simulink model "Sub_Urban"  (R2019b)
settings: Solver=FixedStepAuto  StartTime=0.0  StopTime=3600*24  FixedStep=Tstep  MaxStep=1800  RelTol=1e-3
InitFcn:
  | load('network_parameters')
  | Vnom=400/sqrt(3);
  | Tstep=30*60;
  | MV_LV_transf=0;
StopFcn:
  | run('Simulink_Data.m')
undefined symbols (not defined in the file or in its folder): C_xlpe_185_90, D11, Delta, L_2x16mm, L_2x22mm, L_4x100mm, L_4x16mm, L_4x22mm, L_4x50mm, L_xlpe_185_90, LC, Line_length, R_2x16mm, R_2x22mm, R_4x100mm, R_4x16mm, R_4x22mm, R_4x50mm, R_xlpe_185_90, Source_Voltage
libraries: myLibrary x125, powerlib x89
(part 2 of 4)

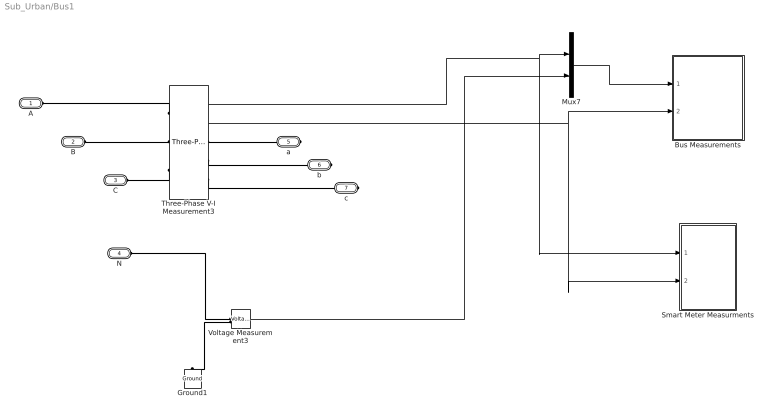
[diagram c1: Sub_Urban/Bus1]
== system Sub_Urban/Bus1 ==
  Bus Measurements : Subsystem
  Ground1 : powerlib/Elements/Ground  LConnTagsString=a
  Mux7 : Mux  Inputs=2
  Smart Meter Measurments : Subsystem
  Three-Phase V-I Measurement3 : powerlib/Measurements/Three-Phase V-I Measurement  VoltageMeasurement=phase-to-ground  SetLabelV=off  LabelV=Vabc  Vpu=off  VpuLL=off  CurrentMeasurement=yes  SetLabelI=off  LabelI=Iabc  Ipu=off  Pbase=100e6  Vbase=500e3  OutputType=Complex  PhasorSimulation=on  PSBequivalent=0
  Voltage Measurement3 : powerlib/Measurements/Voltage Measurement  PhasorSimulation=on  OutputType=Complex  PSBequivalent=0
  A : PMIOPort  Side=Left
  B : PMIOPort  Port=2  Side=Left
  C : PMIOPort  Port=3  Side=Left
  N : PMIOPort  Port=4  Side=Left
  a : PMIOPort  Port=5  Side=Right
  b : PMIOPort  Port=6  Side=Right
  c : PMIOPort  Port=7  Side=Right
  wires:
  Three-Phase V-I Measurement3/2 -> Smart Meter Measurments/2(Iabc), Bus Measurements/2(Iabc)
  Three-Phase V-I Measurement3/1 -> Smart Meter Measurments/1(Vabc), Mux7/1
  Mux7/1 -> Bus Measurements/1(Vabcn)
  Voltage Measurement3/1 -> Mux7/2
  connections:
  Three-Phase V-I Measurement3/LConn1 -- A/RConn1
  Three-Phase V-I Measurement3/LConn3 -- C/RConn1
  Three-Phase V-I Measurement3/LConn2 -- B/RConn1
  Three-Phase V-I Measurement3/RConn1 -- a/RConn1
  Three-Phase V-I Measurement3/RConn2 -- b/RConn1
  Three-Phase V-I Measurement3/RConn3 -- c/RConn1
  Voltage Measurement3/LConn1 -- N/RConn1
  Voltage Measurement3/LConn2 -- Ground1/LConn1

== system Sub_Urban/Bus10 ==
  Constant : Constant  Value=Ph
  Single Phase Load Bus : myLibrary/Single Phase Load Bus  SystemSampleTime=-1  Latency=0  AutoFrameSizeCalculation=off
  To Workspace I : ToWorkspace  VariableName=I10  SaveFormat=Structure With Time  SampleTime=-1
  To Workspace L : ToWorkspace  VariableName=Load5  SaveFormat=Structure With Time  SampleTime=-1
  To Workspace V : ToWorkspace  VariableName=Bus10  SaveFormat=Structure With Time  SampleTime=-1
  Phase : PMIOPort  Tag=PMCPort  Side=Left
  N : PMIOPort  Tag=PMCPort  Port=2  Side=Left
  phase : PMIOPort  Tag=PMCPort  Port=3  Side=Right
  n : PMIOPort  Tag=PMCPort  Port=4  Side=Right
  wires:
  Constant/1 -> Single Phase Load Bus/1
  Single Phase Load Bus/1 -> To Workspace V/1
  Single Phase Load Bus/2 -> To Workspace I/1
  Single Phase Load Bus/3 -> To Workspace L/1
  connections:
  Phase/RConn1 -- Single Phase Load Bus/LConn1
  N/RConn1 -- Single Phase Load Bus/LConn2
  phase/RConn1 -- Single Phase Load Bus/RConn1
  n/RConn1 -- Single Phase Load Bus/RConn2

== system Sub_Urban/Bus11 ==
  Constant : Constant  Value=Ph
  Single Phase Load Bus : myLibrary/Single Phase Load Bus  SystemSampleTime=-1  Latency=0  AutoFrameSizeCalculation=off
  To Workspace I : ToWorkspace  VariableName=I11  SaveFormat=Structure With Time  SampleTime=-1
  To Workspace L : ToWorkspace  VariableName=Load6  SaveFormat=Structure With Time  SampleTime=-1
  To Workspace V : ToWorkspace  VariableName=Bus11  SaveFormat=Structure With Time  SampleTime=-1
  Phase : PMIOPort  Tag=PMCPort  Side=Left
  N : PMIOPort  Tag=PMCPort  Port=2  Side=Left
  phase : PMIOPort  Tag=PMCPort  Port=3  Side=Right
  n : PMIOPort  Tag=PMCPort  Port=4  Side=Right
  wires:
  Constant/1 -> Single Phase Load Bus/1
  Single Phase Load Bus/1 -> To Workspace V/1
  Single Phase Load Bus/2 -> To Workspace I/1
  Single Phase Load Bus/3 -> To Workspace L/1
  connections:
  Phase/RConn1 -- Single Phase Load Bus/LConn1
  N/RConn1 -- Single Phase Load Bus/LConn2
  phase/RConn1 -- Single Phase Load Bus/RConn1
  n/RConn1 -- Single Phase Load Bus/RConn2

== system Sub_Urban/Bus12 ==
  Constant : Constant  Value=Ph
  Single Phase Load Bus : myLibrary/Single Phase Load Bus  SystemSampleTime=-1  Latency=0  AutoFrameSizeCalculation=off
  To Workspace I : ToWorkspace  VariableName=I12  SaveFormat=Structure With Time  SampleTime=-1
  To Workspace L : ToWorkspace  VariableName=Load7  SaveFormat=Structure With Time  SampleTime=-1
  To Workspace V : ToWorkspace  VariableName=Bus12  SaveFormat=Structure With Time  SampleTime=-1
  Phase : PMIOPort  Tag=PMCPort  Side=Left
  N : PMIOPort  Tag=PMCPort  Port=2  Side=Left
  phase : PMIOPort  Tag=PMCPort  Port=3  Side=Right
  n : PMIOPort  Tag=PMCPort  Port=4  Side=Right
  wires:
  Constant/1 -> Single Phase Load Bus/1
  Single Phase Load Bus/1 -> To Workspace V/1
  Single Phase Load Bus/2 -> To Workspace I/1
  Single Phase Load Bus/3 -> To Workspace L/1
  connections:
  Phase/RConn1 -- Single Phase Load Bus/LConn1
  N/RConn1 -- Single Phase Load Bus/LConn2
  phase/RConn1 -- Single Phase Load Bus/RConn1
  n/RConn1 -- Single Phase Load Bus/RConn2

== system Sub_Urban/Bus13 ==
  Constant : Constant  Value=Ph
  Single Phase Load Bus : myLibrary/Single Phase Load Bus  SystemSampleTime=-1  Latency=0  AutoFrameSizeCalculation=off
  To Workspace I : ToWorkspace  VariableName=I13  SaveFormat=Structure With Time  SampleTime=-1
  To Workspace L : ToWorkspace  VariableName=Load8  SaveFormat=Structure With Time  SampleTime=-1
  To Workspace V : ToWorkspace  VariableName=Bus13  SaveFormat=Structure With Time  SampleTime=-1
  Phase : PMIOPort  Tag=PMCPort  Side=Left
  N : PMIOPort  Tag=PMCPort  Port=2  Side=Left
  phase : PMIOPort  Tag=PMCPort  Port=3  Side=Right
  n : PMIOPort  Tag=PMCPort  Port=4  Side=Right
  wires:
  Constant/1 -> Single Phase Load Bus/1
  Single Phase Load Bus/1 -> To Workspace V/1
  Single Phase Load Bus/2 -> To Workspace I/1
  Single Phase Load Bus/3 -> To Workspace L/1
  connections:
  Phase/RConn1 -- Single Phase Load Bus/LConn1
  N/RConn1 -- Single Phase Load Bus/LConn2
  phase/RConn1 -- Single Phase Load Bus/RConn1
  n/RConn1 -- Single Phase Load Bus/RConn2

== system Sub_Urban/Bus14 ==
  Three Phase Zero Bus : myLibrary/Three Phase Zero Bus  SystemSampleTime=-1  Latency=0  AutoFrameSizeCalculation=off
  To Workspace I : ToWorkspace  VariableName=I14  SaveFormat=Structure With Time  SampleTime=-1
  To Workspace V : ToWorkspace  VariableName=Bus14  SaveFormat=Structure With Time  SampleTime=-1
  A : PMIOPort  Tag=PMCPort  Side=Left
  B : PMIOPort  Tag=PMCPort  Port=2  Side=Left
  C : PMIOPort  Tag=PMCPort  Port=3  Side=Left
  N : PMIOPort  Tag=PMCPort  Port=4  Side=Left
  a : PMIOPort  Tag=PMCPort  Port=5  Side=Right
  b : PMIOPort  Tag=PMCPort  Port=6  Side=Right
  c : PMIOPort  Tag=PMCPort  Port=7  Side=Right
  n : PMIOPort  Tag=PMCPort  Port=8  Side=Right
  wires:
  Three Phase Zero Bus/1 -> To Workspace V/1
  Three Phase Zero Bus/2 -> To Workspace I/1
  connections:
  A/RConn1 -- Three Phase Zero Bus/LConn1
  B/RConn1 -- Three Phase Zero Bus/LConn2
  C/RConn1 -- Three Phase Zero Bus/LConn3
  N/RConn1 -- Three Phase Zero Bus/LConn4
  a/RConn1 -- Three Phase Zero Bus/RConn1
  b/RConn1 -- Three Phase Zero Bus/RConn2
  c/RConn1 -- Three Phase Zero Bus/RConn3
  n/RConn1 -- Three Phase Zero Bus/RConn4

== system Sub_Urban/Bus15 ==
  Constant : Constant  Value=Ph
  Single Phase Load Bus : myLibrary/Single Phase Load Bus  SystemSampleTime=-1  Latency=0  AutoFrameSizeCalculation=off
  To Workspace I : ToWorkspace  VariableName=I15  SaveFormat=Structure With Time  SampleTime=-1
  To Workspace L : ToWorkspace  VariableName=Load9  SaveFormat=Structure With Time  SampleTime=-1
  To Workspace V : ToWorkspace  VariableName=Bus15  SaveFormat=Structure With Time  SampleTime=-1
  Phase : PMIOPort  Tag=PMCPort  Side=Left
  N : PMIOPort  Tag=PMCPort  Port=2  Side=Left
  phase : PMIOPort  Tag=PMCPort  Port=3  Side=Right
  n : PMIOPort  Tag=PMCPort  Port=4  Side=Right
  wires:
  Constant/1 -> Single Phase Load Bus/1
  Single Phase Load Bus/1 -> To Workspace V/1
  Single Phase Load Bus/2 -> To Workspace I/1
  Single Phase Load Bus/3 -> To Workspace L/1
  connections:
  Phase/RConn1 -- Single Phase Load Bus/LConn1
  N/RConn1 -- Single Phase Load Bus/LConn2
  phase/RConn1 -- Single Phase Load Bus/RConn1
  n/RConn1 -- Single Phase Load Bus/RConn2

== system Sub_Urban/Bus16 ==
  Three Phase Zero Bus : myLibrary/Three Phase Zero Bus  SystemSampleTime=-1  Latency=0  AutoFrameSizeCalculation=off
  To Workspace I : ToWorkspace  VariableName=I16  SaveFormat=Structure With Time  SampleTime=-1
  To Workspace V : ToWorkspace  VariableName=Bus16  SaveFormat=Structure With Time  SampleTime=-1
  A : PMIOPort  Tag=PMCPort  Side=Left
  B : PMIOPort  Tag=PMCPort  Port=2  Side=Left
  C : PMIOPort  Tag=PMCPort  Port=3  Side=Left
  N : PMIOPort  Tag=PMCPort  Port=4  Side=Left
  a : PMIOPort  Tag=PMCPort  Port=5  Side=Right
  b : PMIOPort  Tag=PMCPort  Port=6  Side=Right
  c : PMIOPort  Tag=PMCPort  Port=7  Side=Right
  n : PMIOPort  Tag=PMCPort  Port=8  Side=Right
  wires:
  Three Phase Zero Bus/1 -> To Workspace V/1
  Three Phase Zero Bus/2 -> To Workspace I/1
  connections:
  A/RConn1 -- Three Phase Zero Bus/LConn1
  B/RConn1 -- Three Phase Zero Bus/LConn2
  C/RConn1 -- Three Phase Zero Bus/LConn3
  N/RConn1 -- Three Phase Zero Bus/LConn4
  a/RConn1 -- Three Phase Zero Bus/RConn1
  b/RConn1 -- Three Phase Zero Bus/RConn2
  c/RConn1 -- Three Phase Zero Bus/RConn3
  n/RConn1 -- Three Phase Zero Bus/RConn4

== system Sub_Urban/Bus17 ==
  Constant : Constant  Value=Ph
  Single Phase Load Bus : myLibrary/Single Phase Load Bus  SystemSampleTime=-1  Latency=0  AutoFrameSizeCalculation=off
  To Workspace I : ToWorkspace  VariableName=I17  SaveFormat=Structure With Time  SampleTime=-1
  To Workspace L : ToWorkspace  VariableName=Load10  SaveFormat=Structure With Time  SampleTime=-1
  To Workspace V : ToWorkspace  VariableName=Bus17  SaveFormat=Structure With Time  SampleTime=-1
  Phase : PMIOPort  Tag=PMCPort  Side=Left
  N : PMIOPort  Tag=PMCPort  Port=2  Side=Left
  phase : PMIOPort  Tag=PMCPort  Port=3  Side=Right
  n : PMIOPort  Tag=PMCPort  Port=4  Side=Right
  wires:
  Constant/1 -> Single Phase Load Bus/1
  Single Phase Load Bus/1 -> To Workspace V/1
  Single Phase Load Bus/2 -> To Workspace I/1
  Single Phase Load Bus/3 -> To Workspace L/1
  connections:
  Phase/RConn1 -- Single Phase Load Bus/LConn1
  N/RConn1 -- Single Phase Load Bus/LConn2
  phase/RConn1 -- Single Phase Load Bus/RConn1
  n/RConn1 -- Single Phase Load Bus/RConn2

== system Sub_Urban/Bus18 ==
  Constant : Constant  Value=Ph
  Single Phase Load Bus : myLibrary/Single Phase Load Bus  SystemSampleTime=-1  Latency=0  AutoFrameSizeCalculation=off
  To Workspace I : ToWorkspace  VariableName=I18  SaveFormat=Structure With Time  SampleTime=-1
  To Workspace L : ToWorkspace  VariableName=Load11  SaveFormat=Structure With Time  SampleTime=-1
  To Workspace V : ToWorkspace  VariableName=Bus18  SaveFormat=Structure With Time  SampleTime=-1
  Phase : PMIOPort  Tag=PMCPort  Side=Left
  N : PMIOPort  Tag=PMCPort  Port=2  Side=Left
  phase : PMIOPort  Tag=PMCPort  Port=3  Side=Right
  n : PMIOPort  Tag=PMCPort  Port=4  Side=Right
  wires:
  Constant/1 -> Single Phase Load Bus/1
  Single Phase Load Bus/1 -> To Workspace V/1
  Single Phase Load Bus/2 -> To Workspace I/1
  Single Phase Load Bus/3 -> To Workspace L/1
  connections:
  Phase/RConn1 -- Single Phase Load Bus/LConn1
  N/RConn1 -- Single Phase Load Bus/LConn2
  phase/RConn1 -- Single Phase Load Bus/RConn1
  n/RConn1 -- Single Phase Load Bus/RConn2

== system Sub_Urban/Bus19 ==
  Constant : Constant  Value=Ph
  Single Phase Load Bus : myLibrary/Single Phase Load Bus  SystemSampleTime=-1  Latency=0  AutoFrameSizeCalculation=off
  To Workspace I : ToWorkspace  VariableName=I19  SaveFormat=Structure With Time  SampleTime=-1
  To Workspace L : ToWorkspace  VariableName=Load12  SaveFormat=Structure With Time  SampleTime=-1
  To Workspace V : ToWorkspace  VariableName=Bus19  SaveFormat=Structure With Time  SampleTime=-1
  Phase : PMIOPort  Tag=PMCPort  Side=Left
  N : PMIOPort  Tag=PMCPort  Port=2  Side=Left
  phase : PMIOPort  Tag=PMCPort  Port=3  Side=Right
  n : PMIOPort  Tag=PMCPort  Port=4  Side=Right
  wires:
  Constant/1 -> Single Phase Load Bus/1
  Single Phase Load Bus/1 -> To Workspace V/1
  Single Phase Load Bus/2 -> To Workspace I/1
  Single Phase Load Bus/3 -> To Workspace L/1
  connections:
  Phase/RConn1 -- Single Phase Load Bus/LConn1
  N/RConn1 -- Single Phase Load Bus/LConn2
  phase/RConn1 -- Single Phase Load Bus/RConn1
  n/RConn1 -- Single Phase Load Bus/RConn2

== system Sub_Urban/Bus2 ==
  Three Phase Zero Bus : myLibrary/Three Phase Zero Bus  SystemSampleTime=-1  Latency=0  AutoFrameSizeCalculation=off
  To Workspace I : ToWorkspace  VariableName=I2  SaveFormat=Structure With Time  SampleTime=-1
  To Workspace V : ToWorkspace  VariableName=Bus2  SaveFormat=Structure With Time  SampleTime=-1
  A : PMIOPort  Tag=PMCPort  Side=Left
  B : PMIOPort  Tag=PMCPort  Port=2  Side=Left
  C : PMIOPort  Tag=PMCPort  Port=3  Side=Left
  N : PMIOPort  Tag=PMCPort  Port=4  Side=Left
  a : PMIOPort  Tag=PMCPort  Port=5  Side=Right
  b : PMIOPort  Tag=PMCPort  Port=6  Side=Right
  c : PMIOPort  Tag=PMCPort  Port=7  Side=Right
  n : PMIOPort  Tag=PMCPort  Port=8  Side=Right
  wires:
  Three Phase Zero Bus/1 -> To Workspace V/1
  Three Phase Zero Bus/2 -> To Workspace I/1
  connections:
  Three Phase Zero Bus/LConn1 -- A/RConn1
  Three Phase Zero Bus/LConn2 -- B/RConn1
  Three Phase Zero Bus/LConn3 -- C/RConn1
  Three Phase Zero Bus/LConn4 -- N/RConn1
  Three Phase Zero Bus/RConn1 -- a/RConn1
  Three Phase Zero Bus/RConn2 -- b/RConn1
  Three Phase Zero Bus/RConn3 -- c/RConn1
  n/RConn1 -- Three Phase Zero Bus/RConn4

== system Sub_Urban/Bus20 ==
  Three Phase Zero Bus : myLibrary/Three Phase Zero Bus  SystemSampleTime=-1  Latency=0  AutoFrameSizeCalculation=off
  To Workspace I : ToWorkspace  VariableName=I20  SaveFormat=Structure With Time  SampleTime=-1
  To Workspace V : ToWorkspace  VariableName=Bus20  SaveFormat=Structure With Time  SampleTime=-1
  A : PMIOPort  Tag=PMCPort  Side=Left
  B : PMIOPort  Tag=PMCPort  Port=2  Side=Left
  C : PMIOPort  Tag=PMCPort  Port=3  Side=Left
  N : PMIOPort  Tag=PMCPort  Port=4  Side=Left
  a : PMIOPort  Tag=PMCPort  Port=5  Side=Right
  b : PMIOPort  Tag=PMCPort  Port=6  Side=Right
  c : PMIOPort  Tag=PMCPort  Port=7  Side=Right
  n : PMIOPort  Tag=PMCPort  Port=8  Side=Right
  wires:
  Three Phase Zero Bus/1 -> To Workspace V/1
  Three Phase Zero Bus/2 -> To Workspace I/1
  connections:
  A/RConn1 -- Three Phase Zero Bus/LConn1
  B/RConn1 -- Three Phase Zero Bus/LConn2
  C/RConn1 -- Three Phase Zero Bus/LConn3
  N/RConn1 -- Three Phase Zero Bus/LConn4
  a/RConn1 -- Three Phase Zero Bus/RConn1
  b/RConn1 -- Three Phase Zero Bus/RConn2
  c/RConn1 -- Three Phase Zero Bus/RConn3
  n/RConn1 -- Three Phase Zero Bus/RConn4

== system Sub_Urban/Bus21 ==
  Constant : Constant  Value=Ph
  Single Phase Load Bus : myLibrary/Single Phase Load Bus  SystemSampleTime=-1  Latency=0  AutoFrameSizeCalculation=off
  To Workspace I : ToWorkspace  VariableName=I21  SaveFormat=Structure With Time  SampleTime=-1
  To Workspace L : ToWorkspace  VariableName=Load13  SaveFormat=Structure With Time  SampleTime=-1
  To Workspace V : ToWorkspace  VariableName=Bus21  SaveFormat=Structure With Time  SampleTime=-1
  Phase : PMIOPort  Tag=PMCPort  Side=Left
  N : PMIOPort  Tag=PMCPort  Port=2  Side=Left
  phase : PMIOPort  Tag=PMCPort  Port=3  Side=Right
  n : PMIOPort  Tag=PMCPort  Port=4  Side=Right
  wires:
  Constant/1 -> Single Phase Load Bus/1
  Single Phase Load Bus/1 -> To Workspace V/1
  Single Phase Load Bus/2 -> To Workspace I/1
  Single Phase Load Bus/3 -> To Workspace L/1
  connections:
  Phase/RConn1 -- Single Phase Load Bus/LConn1
  N/RConn1 -- Single Phase Load Bus/LConn2
  phase/RConn1 -- Single Phase Load Bus/RConn1
  n/RConn1 -- Single Phase Load Bus/RConn2

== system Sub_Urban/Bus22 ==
  Three Phase Zero Bus : myLibrary/Three Phase Zero Bus  SystemSampleTime=-1  Latency=0  AutoFrameSizeCalculation=off
  To Workspace I : ToWorkspace  VariableName=I22  SaveFormat=Structure With Time  SampleTime=-1
  To Workspace V : ToWorkspace  VariableName=Bus22  SaveFormat=Structure With Time  SampleTime=-1
  A : PMIOPort  Tag=PMCPort  Side=Left
  B : PMIOPort  Tag=PMCPort  Port=2  Side=Left
  C : PMIOPort  Tag=PMCPort  Port=3  Side=Left
  N : PMIOPort  Tag=PMCPort  Port=4  Side=Left
  a : PMIOPort  Tag=PMCPort  Port=5  Side=Right
  b : PMIOPort  Tag=PMCPort  Port=6  Side=Right
  c : PMIOPort  Tag=PMCPort  Port=7  Side=Right
  n : PMIOPort  Tag=PMCPort  Port=8  Side=Right
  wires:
  Three Phase Zero Bus/1 -> To Workspace V/1
  Three Phase Zero Bus/2 -> To Workspace I/1
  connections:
  A/RConn1 -- Three Phase Zero Bus/LConn1
  B/RConn1 -- Three Phase Zero Bus/LConn2
  C/RConn1 -- Three Phase Zero Bus/LConn3
  N/RConn1 -- Three Phase Zero Bus/LConn4
  a/RConn1 -- Three Phase Zero Bus/RConn1
  b/RConn1 -- Three Phase Zero Bus/RConn2
  c/RConn1 -- Three Phase Zero Bus/RConn3
  n/RConn1 -- Three Phase Zero Bus/RConn4

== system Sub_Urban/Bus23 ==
  Constant : Constant  Value=Ph
  Single Phase Load Bus : myLibrary/Single Phase Load Bus  SystemSampleTime=-1  Latency=0  AutoFrameSizeCalculation=off
  To Workspace I : ToWorkspace  VariableName=I23  SaveFormat=Structure With Time  SampleTime=-1
  To Workspace L : ToWorkspace  VariableName=Load14  SaveFormat=Structure With Time  SampleTime=-1
  To Workspace V : ToWorkspace  VariableName=Bus23  SaveFormat=Structure With Time  SampleTime=-1
  Phase : PMIOPort  Tag=PMCPort  Side=Left
  N : PMIOPort  Tag=PMCPort  Port=2  Side=Left
  phase : PMIOPort  Tag=PMCPort  Port=3  Side=Right
  n : PMIOPort  Tag=PMCPort  Port=4  Side=Right
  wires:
  Constant/1 -> Single Phase Load Bus/1
  Single Phase Load Bus/1 -> To Workspace V/1
  Single Phase Load Bus/2 -> To Workspace I/1
  Single Phase Load Bus/3 -> To Workspace L/1
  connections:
  Phase/RConn1 -- Single Phase Load Bus/LConn1
  N/RConn1 -- Single Phase Load Bus/LConn2
  phase/RConn1 -- Single Phase Load Bus/RConn1
  n/RConn1 -- Single Phase Load Bus/RConn2

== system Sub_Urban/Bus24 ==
  Constant : Constant  Value=Ph
  Single Phase Load Bus : myLibrary/Single Phase Load Bus  SystemSampleTime=-1  Latency=0  AutoFrameSizeCalculation=off
  To Workspace I : ToWorkspace  VariableName=I24  SaveFormat=Structure With Time  SampleTime=-1
  To Workspace L : ToWorkspace  VariableName=Load15  SaveFormat=Structure With Time  SampleTime=-1
  To Workspace V : ToWorkspace  VariableName=Bus24  SaveFormat=Structure With Time  SampleTime=-1
  Phase : PMIOPort  Tag=PMCPort  Side=Left
  N : PMIOPort  Tag=PMCPort  Port=2  Side=Left
  phase : PMIOPort  Tag=PMCPort  Port=3  Side=Right
  n : PMIOPort  Tag=PMCPort  Port=4  Side=Right
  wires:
  Constant/1 -> Single Phase Load Bus/1
  Single Phase Load Bus/1 -> To Workspace V/1
  Single Phase Load Bus/2 -> To Workspace I/1
  Single Phase Load Bus/3 -> To Workspace L/1
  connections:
  Phase/RConn1 -- Single Phase Load Bus/LConn1
  N/RConn1 -- Single Phase Load Bus/LConn2
  phase/RConn1 -- Single Phase Load Bus/RConn1
  n/RConn1 -- Single Phase Load Bus/RConn2

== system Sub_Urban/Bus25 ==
  Three Phase Zero Bus : myLibrary/Three Phase Zero Bus  SystemSampleTime=-1  Latency=0  AutoFrameSizeCalculation=off
  To Workspace I : ToWorkspace  VariableName=I25  SaveFormat=Structure With Time  SampleTime=-1
  To Workspace V : ToWorkspace  VariableName=Bus25  SaveFormat=Structure With Time  SampleTime=-1
  A : PMIOPort  Tag=PMCPort  Side=Left
  B : PMIOPort  Tag=PMCPort  Port=2  Side=Left
  C : PMIOPort  Tag=PMCPort  Port=3  Side=Left
  N : PMIOPort  Tag=PMCPort  Port=4  Side=Left
  a : PMIOPort  Tag=PMCPort  Port=5  Side=Right
  b : PMIOPort  Tag=PMCPort  Port=6  Side=Right
  c : PMIOPort  Tag=PMCPort  Port=7  Side=Right
  n : PMIOPort  Tag=PMCPort  Port=8  Side=Right
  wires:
  Three Phase Zero Bus/1 -> To Workspace V/1
  Three Phase Zero Bus/2 -> To Workspace I/1
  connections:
  A/RConn1 -- Three Phase Zero Bus/LConn1
  B/RConn1 -- Three Phase Zero Bus/LConn2
  C/RConn1 -- Three Phase Zero Bus/LConn3
  N/RConn1 -- Three Phase Zero Bus/LConn4
  a/RConn1 -- Three Phase Zero Bus/RConn1
  b/RConn1 -- Three Phase Zero Bus/RConn2
  c/RConn1 -- Three Phase Zero Bus/RConn3
  n/RConn1 -- Three Phase Zero Bus/RConn4

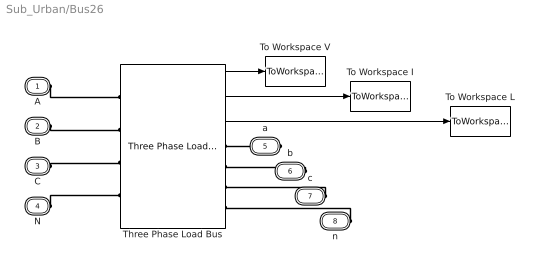
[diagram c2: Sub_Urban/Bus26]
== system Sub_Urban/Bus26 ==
  Three Phase Load Bus : myLibrary/Three Phase Load Bus  SystemSampleTime=-1  Latency=0  AutoFrameSizeCalculation=off
  To Workspace I : ToWorkspace  VariableName=I26  SaveFormat=Structure With Time  SampleTime=-1
  To Workspace L : ToWorkspace  VariableName=Load16  SaveFormat=Structure With Time  SampleTime=-1
  To Workspace V : ToWorkspace  VariableName=Bus26  SaveFormat=Structure With Time  SampleTime=-1
  A : PMIOPort  Tag=PMCPort  Side=Left
  B : PMIOPort  Tag=PMCPort  Port=2  Side=Left
  C : PMIOPort  Tag=PMCPort  Port=3  Side=Left
  N : PMIOPort  Tag=PMCPort  Port=4  Side=Left
  a : PMIOPort  Tag=PMCPort  Port=5  Side=Right
  b : PMIOPort  Tag=PMCPort  Port=6  Side=Right
  c : PMIOPort  Tag=PMCPort  Port=7  Side=Right
  n : PMIOPort  Tag=PMCPort  Port=8  Side=Right
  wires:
  Three Phase Load Bus/1 -> To Workspace V/1
  Three Phase Load Bus/2 -> To Workspace I/1
  Three Phase Load Bus/3 -> To Workspace L/1
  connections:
  N/RConn1 -- Three Phase Load Bus/LConn4
  C/RConn1 -- Three Phase Load Bus/LConn3
  n/RConn1 -- Three Phase Load Bus/RConn4
  B/RConn1 -- Three Phase Load Bus/LConn2
  A/RConn1 -- Three Phase Load Bus/LConn1
  b/RConn1 -- Three Phase Load Bus/RConn2
  c/RConn1 -- Three Phase Load Bus/RConn3
  a/RConn1 -- Three Phase Load Bus/RConn1

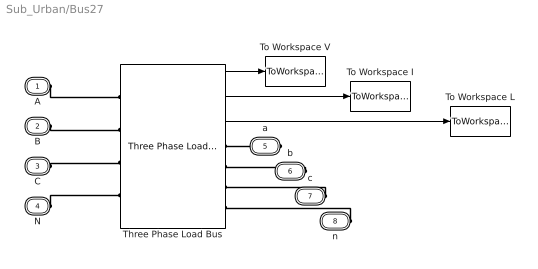
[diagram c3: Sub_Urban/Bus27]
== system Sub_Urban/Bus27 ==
  Three Phase Load Bus : myLibrary/Three Phase Load Bus  SystemSampleTime=-1  Latency=0  AutoFrameSizeCalculation=off
  To Workspace I : ToWorkspace  VariableName=I27  SaveFormat=Structure With Time  SampleTime=-1
  To Workspace L : ToWorkspace  VariableName=Load17  SaveFormat=Structure With Time  SampleTime=-1
  To Workspace V : ToWorkspace  VariableName=Bus27  SaveFormat=Structure With Time  SampleTime=-1
  A : PMIOPort  Tag=PMCPort  Side=Left
  B : PMIOPort  Tag=PMCPort  Port=2  Side=Left
  C : PMIOPort  Tag=PMCPort  Port=3  Side=Left
  N : PMIOPort  Tag=PMCPort  Port=4  Side=Left
  a : PMIOPort  Tag=PMCPort  Port=5  Side=Right
  b : PMIOPort  Tag=PMCPort  Port=6  Side=Right
  c : PMIOPort  Tag=PMCPort  Port=7  Side=Right
  n : PMIOPort  Tag=PMCPort  Port=8  Side=Right
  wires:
  Three Phase Load Bus/1 -> To Workspace V/1
  Three Phase Load Bus/2 -> To Workspace I/1
  Three Phase Load Bus/3 -> To Workspace L/1
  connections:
  N/RConn1 -- Three Phase Load Bus/LConn4
  C/RConn1 -- Three Phase Load Bus/LConn3
  n/RConn1 -- Three Phase Load Bus/RConn4
  B/RConn1 -- Three Phase Load Bus/LConn2
  A/RConn1 -- Three Phase Load Bus/LConn1
  b/RConn1 -- Three Phase Load Bus/RConn2
  c/RConn1 -- Three Phase Load Bus/RConn3
  a/RConn1 -- Three Phase Load Bus/RConn1

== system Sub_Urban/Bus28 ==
  Constant : Constant  Value=Ph
  Single Phase Load Bus : myLibrary/Single Phase Load Bus  SystemSampleTime=-1  Latency=0  AutoFrameSizeCalculation=off
  To Workspace I : ToWorkspace  VariableName=I28  SaveFormat=Structure With Time  SampleTime=-1
  To Workspace L : ToWorkspace  VariableName=Load18  SaveFormat=Structure With Time  SampleTime=-1
  To Workspace V : ToWorkspace  VariableName=Bus28  SaveFormat=Structure With Time  SampleTime=-1
  Phase : PMIOPort  Tag=PMCPort  Side=Left
  N : PMIOPort  Tag=PMCPort  Port=2  Side=Left
  phase : PMIOPort  Tag=PMCPort  Port=3  Side=Right
  n : PMIOPort  Tag=PMCPort  Port=4  Side=Right
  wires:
  Constant/1 -> Single Phase Load Bus/1
  Single Phase Load Bus/1 -> To Workspace V/1
  Single Phase Load Bus/2 -> To Workspace I/1
  Single Phase Load Bus/3 -> To Workspace L/1
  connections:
  Phase/RConn1 -- Single Phase Load Bus/LConn1
  N/RConn1 -- Single Phase Load Bus/LConn2
  phase/RConn1 -- Single Phase Load Bus/RConn1
  n/RConn1 -- Single Phase Load Bus/RConn2

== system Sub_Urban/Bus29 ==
  Constant : Constant  Value=Ph
  Single Phase Load Bus : myLibrary/Single Phase Load Bus  SystemSampleTime=-1  Latency=0  AutoFrameSizeCalculation=off
  To Workspace I : ToWorkspace  VariableName=I29  SaveFormat=Structure With Time  SampleTime=-1
  To Workspace L : ToWorkspace  VariableName=Load19  SaveFormat=Structure With Time  SampleTime=-1
  To Workspace V : ToWorkspace  VariableName=Bus29  SaveFormat=Structure With Time  SampleTime=-1
  Phase : PMIOPort  Tag=PMCPort  Side=Left
  N : PMIOPort  Tag=PMCPort  Port=2  Side=Left
  phase : PMIOPort  Tag=PMCPort  Port=3  Side=Right
  n : PMIOPort  Tag=PMCPort  Port=4  Side=Right
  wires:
  Constant/1 -> Single Phase Load Bus/1
  Single Phase Load Bus/1 -> To Workspace V/1
  Single Phase Load Bus/2 -> To Workspace I/1
  Single Phase Load Bus/3 -> To Workspace L/1
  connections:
  Phase/RConn1 -- Single Phase Load Bus/LConn1
  N/RConn1 -- Single Phase Load Bus/LConn2
  phase/RConn1 -- Single Phase Load Bus/RConn1
  n/RConn1 -- Single Phase Load Bus/RConn2

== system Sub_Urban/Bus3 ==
  Three Phase Zero Bus : myLibrary/Three Phase Zero Bus  SystemSampleTime=-1  Latency=0  AutoFrameSizeCalculation=off
  To Workspace I : ToWorkspace  VariableName=I3  SaveFormat=Structure With Time  SampleTime=-1
  To Workspace V : ToWorkspace  VariableName=Bus3  SaveFormat=Structure With Time  SampleTime=-1
  A : PMIOPort  Tag=PMCPort  Side=Left
  B : PMIOPort  Tag=PMCPort  Port=2  Side=Left
  C : PMIOPort  Tag=PMCPort  Port=3  Side=Left
  N : PMIOPort  Tag=PMCPort  Port=4  Side=Left
  a : PMIOPort  Tag=PMCPort  Port=5  Side=Right
  b : PMIOPort  Tag=PMCPort  Port=6  Side=Right
  c : PMIOPort  Tag=PMCPort  Port=7  Side=Right
  n : PMIOPort  Tag=PMCPort  Port=8  Side=Right
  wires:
  Three Phase Zero Bus/1 -> To Workspace V/1
  Three Phase Zero Bus/2 -> To Workspace I/1
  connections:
  A/RConn1 -- Three Phase Zero Bus/LConn1
  B/RConn1 -- Three Phase Zero Bus/LConn2
  C/RConn1 -- Three Phase Zero Bus/LConn3
  N/RConn1 -- Three Phase Zero Bus/LConn4
  a/RConn1 -- Three Phase Zero Bus/RConn1
  b/RConn1 -- Three Phase Zero Bus/RConn2
  c/RConn1 -- Three Phase Zero Bus/RConn3
  n/RConn1 -- Three Phase Zero Bus/RConn4

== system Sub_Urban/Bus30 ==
  Three Phase Zero Bus : myLibrary/Three Phase Zero Bus  SystemSampleTime=-1  Latency=0  AutoFrameSizeCalculation=off
  To Workspace I : ToWorkspace  VariableName=I30  SaveFormat=Structure With Time  SampleTime=-1
  To Workspace V : ToWorkspace  VariableName=Bus30  SaveFormat=Structure With Time  SampleTime=-1
  A : PMIOPort  Tag=PMCPort  Side=Left
  B : PMIOPort  Tag=PMCPort  Port=2  Side=Left
  C : PMIOPort  Tag=PMCPort  Port=3  Side=Left
  N : PMIOPort  Tag=PMCPort  Port=4  Side=Left
  a : PMIOPort  Tag=PMCPort  Port=5  Side=Right
  b : PMIOPort  Tag=PMCPort  Port=6  Side=Right
  c : PMIOPort  Tag=PMCPort  Port=7  Side=Right
  n : PMIOPort  Tag=PMCPort  Port=8  Side=Right
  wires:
  Three Phase Zero Bus/1 -> To Workspace V/1
  Three Phase Zero Bus/2 -> To Workspace I/1
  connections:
  A/RConn1 -- Three Phase Zero Bus/LConn1
  B/RConn1 -- Three Phase Zero Bus/LConn2
  C/RConn1 -- Three Phase Zero Bus/LConn3
  N/RConn1 -- Three Phase Zero Bus/LConn4
  a/RConn1 -- Three Phase Zero Bus/RConn1
  b/RConn1 -- Three Phase Zero Bus/RConn2
  c/RConn1 -- Three Phase Zero Bus/RConn3
  n/RConn1 -- Three Phase Zero Bus/RConn4

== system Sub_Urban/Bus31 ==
  Three Phase Zero Bus : myLibrary/Three Phase Zero Bus  SystemSampleTime=-1  Latency=0  AutoFrameSizeCalculation=off
  To Workspace I : ToWorkspace  VariableName=I31  SaveFormat=Structure With Time  SampleTime=-1
  To Workspace V : ToWorkspace  VariableName=Bus31  SaveFormat=Structure With Time  SampleTime=-1
  A : PMIOPort  Tag=PMCPort  Side=Left
  B : PMIOPort  Tag=PMCPort  Port=2  Side=Left
  C : PMIOPort  Tag=PMCPort  Port=3  Side=Left
  N : PMIOPort  Tag=PMCPort  Port=4  Side=Left
  a : PMIOPort  Tag=PMCPort  Port=5  Side=Right
  b : PMIOPort  Tag=PMCPort  Port=6  Side=Right
  c : PMIOPort  Tag=PMCPort  Port=7  Side=Right
  n : PMIOPort  Tag=PMCPort  Port=8  Side=Right
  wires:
  Three Phase Zero Bus/1 -> To Workspace V/1
  Three Phase Zero Bus/2 -> To Workspace I/1
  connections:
  A/RConn1 -- Three Phase Zero Bus/LConn1
  B/RConn1 -- Three Phase Zero Bus/LConn2
  C/RConn1 -- Three Phase Zero Bus/LConn3
  N/RConn1 -- Three Phase Zero Bus/LConn4
  a/RConn1 -- Three Phase Zero Bus/RConn1
  b/RConn1 -- Three Phase Zero Bus/RConn2
  c/RConn1 -- Three Phase Zero Bus/RConn3
  n/RConn1 -- Three Phase Zero Bus/RConn4

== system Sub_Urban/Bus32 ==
  Constant : Constant  Value=Ph
  Single Phase Load Bus : myLibrary/Single Phase Load Bus  SystemSampleTime=-1  Latency=0  AutoFrameSizeCalculation=off
  To Workspace I : ToWorkspace  VariableName=I32  SaveFormat=Structure With Time  SampleTime=-1
  To Workspace L : ToWorkspace  VariableName=Load20  SaveFormat=Structure With Time  SampleTime=-1
  To Workspace V : ToWorkspace  VariableName=Bus32  SaveFormat=Structure With Time  SampleTime=-1
  Phase : PMIOPort  Tag=PMCPort  Side=Left
  N : PMIOPort  Tag=PMCPort  Port=2  Side=Left
  phase : PMIOPort  Tag=PMCPort  Port=3  Side=Right
  n : PMIOPort  Tag=PMCPort  Port=4  Side=Right
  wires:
  Constant/1 -> Single Phase Load Bus/1
  Single Phase Load Bus/1 -> To Workspace V/1
  Single Phase Load Bus/2 -> To Workspace I/1
  Single Phase Load Bus/3 -> To Workspace L/1
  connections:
  Phase/RConn1 -- Single Phase Load Bus/LConn1
  N/RConn1 -- Single Phase Load Bus/LConn2
  phase/RConn1 -- Single Phase Load Bus/RConn1
  n/RConn1 -- Single Phase Load Bus/RConn2

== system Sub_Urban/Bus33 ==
  Three Phase Zero Bus : myLibrary/Three Phase Zero Bus  SystemSampleTime=-1  Latency=0  AutoFrameSizeCalculation=off
  To Workspace I : ToWorkspace  VariableName=I33  SaveFormat=Structure With Time  SampleTime=-1
  To Workspace V : ToWorkspace  VariableName=Bus33  SaveFormat=Structure With Time  SampleTime=-1
  A : PMIOPort  Tag=PMCPort  Side=Left
  B : PMIOPort  Tag=PMCPort  Port=2  Side=Left
  C : PMIOPort  Tag=PMCPort  Port=3  Side=Left
  N : PMIOPort  Tag=PMCPort  Port=4  Side=Left
  a : PMIOPort  Tag=PMCPort  Port=5  Side=Right
  b : PMIOPort  Tag=PMCPort  Port=6  Side=Right
  c : PMIOPort  Tag=PMCPort  Port=7  Side=Right
  n : PMIOPort  Tag=PMCPort  Port=8  Side=Right
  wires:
  Three Phase Zero Bus/1 -> To Workspace V/1
  Three Phase Zero Bus/2 -> To Workspace I/1
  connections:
  A/RConn1 -- Three Phase Zero Bus/LConn1
  B/RConn1 -- Three Phase Zero Bus/LConn2
  C/RConn1 -- Three Phase Zero Bus/LConn3
  N/RConn1 -- Three Phase Zero Bus/LConn4
  a/RConn1 -- Three Phase Zero Bus/RConn1
  b/RConn1 -- Three Phase Zero Bus/RConn2
  c/RConn1 -- Three Phase Zero Bus/RConn3
  n/RConn1 -- Three Phase Zero Bus/RConn4

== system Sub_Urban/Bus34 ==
  Constant : Constant  Value=Ph
  Single Phase Load Bus : myLibrary/Single Phase Load Bus  SystemSampleTime=-1  Latency=0  AutoFrameSizeCalculation=off
  To Workspace I : ToWorkspace  VariableName=I34  SaveFormat=Structure With Time  SampleTime=-1
  To Workspace L : ToWorkspace  VariableName=Load21  SaveFormat=Structure With Time  SampleTime=-1
  To Workspace V : ToWorkspace  VariableName=Bus34  SaveFormat=Structure With Time  SampleTime=-1
  Phase : PMIOPort  Tag=PMCPort  Side=Left
  N : PMIOPort  Tag=PMCPort  Port=2  Side=Left
  phase : PMIOPort  Tag=PMCPort  Port=3  Side=Right
  n : PMIOPort  Tag=PMCPort  Port=4  Side=Right
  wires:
  Constant/1 -> Single Phase Load Bus/1
  Single Phase Load Bus/1 -> To Workspace V/1
  Single Phase Load Bus/2 -> To Workspace I/1
  Single Phase Load Bus/3 -> To Workspace L/1
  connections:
  Phase/RConn1 -- Single Phase Load Bus/LConn1
  N/RConn1 -- Single Phase Load Bus/LConn2
  phase/RConn1 -- Single Phase Load Bus/RConn1
  n/RConn1 -- Single Phase Load Bus/RConn2

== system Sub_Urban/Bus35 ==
  Constant : Constant  Value=Ph
  Single Phase Load Bus : myLibrary/Single Phase Load Bus  SystemSampleTime=-1  Latency=0  AutoFrameSizeCalculation=off
  To Workspace I : ToWorkspace  VariableName=I35  SaveFormat=Structure With Time  SampleTime=-1
  To Workspace L : ToWorkspace  VariableName=Load22  SaveFormat=Structure With Time  SampleTime=-1
  To Workspace V : ToWorkspace  VariableName=Bus35  SaveFormat=Structure With Time  SampleTime=-1
  Phase : PMIOPort  Tag=PMCPort  Side=Left
  N : PMIOPort  Tag=PMCPort  Port=2  Side=Left
  phase : PMIOPort  Tag=PMCPort  Port=3  Side=Right
  n : PMIOPort  Tag=PMCPort  Port=4  Side=Right
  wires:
  Constant/1 -> Single Phase Load Bus/1
  Single Phase Load Bus/1 -> To Workspace V/1
  Single Phase Load Bus/2 -> To Workspace I/1
  Single Phase Load Bus/3 -> To Workspace L/1
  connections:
  Phase/RConn1 -- Single Phase Load Bus/LConn1
  N/RConn1 -- Single Phase Load Bus/LConn2
  phase/RConn1 -- Single Phase Load Bus/RConn1
  n/RConn1 -- Single Phase Load Bus/RConn2

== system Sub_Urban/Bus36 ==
  Constant : Constant  Value=Ph
  Single Phase Load Bus : myLibrary/Single Phase Load Bus  SystemSampleTime=-1  Latency=0  AutoFrameSizeCalculation=off
  To Workspace I : ToWorkspace  VariableName=I36  SaveFormat=Structure With Time  SampleTime=-1
  To Workspace L : ToWorkspace  VariableName=Load23  SaveFormat=Structure With Time  SampleTime=-1
  To Workspace V : ToWorkspace  VariableName=Bus36  SaveFormat=Structure With Time  SampleTime=-1
  Phase : PMIOPort  Tag=PMCPort  Side=Left
  N : PMIOPort  Tag=PMCPort  Port=2  Side=Left
  phase : PMIOPort  Tag=PMCPort  Port=3  Side=Right
  n : PMIOPort  Tag=PMCPort  Port=4  Side=Right
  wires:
  Constant/1 -> Single Phase Load Bus/1
  Single Phase Load Bus/1 -> To Workspace V/1
  Single Phase Load Bus/2 -> To Workspace I/1
  Single Phase Load Bus/3 -> To Workspace L/1
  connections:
  Phase/RConn1 -- Single Phase Load Bus/LConn1
  N/RConn1 -- Single Phase Load Bus/LConn2
  phase/RConn1 -- Single Phase Load Bus/RConn1
  n/RConn1 -- Single Phase Load Bus/RConn2

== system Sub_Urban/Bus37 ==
  Constant : Constant  Value=Ph
  Single Phase Load Bus : myLibrary/Single Phase Load Bus  SystemSampleTime=-1  Latency=0  AutoFrameSizeCalculation=off
  To Workspace I : ToWorkspace  VariableName=I37  SaveFormat=Structure With Time  SampleTime=-1
  To Workspace L : ToWorkspace  VariableName=Load24  SaveFormat=Structure With Time  SampleTime=-1
  To Workspace V : ToWorkspace  VariableName=Bus37  SaveFormat=Structure With Time  SampleTime=-1
  Phase : PMIOPort  Tag=PMCPort  Side=Left
  N : PMIOPort  Tag=PMCPort  Port=2  Side=Left
  phase : PMIOPort  Tag=PMCPort  Port=3  Side=Right
  n : PMIOPort  Tag=PMCPort  Port=4  Side=Right
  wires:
  Constant/1 -> Single Phase Load Bus/1
  Single Phase Load Bus/1 -> To Workspace V/1
  Single Phase Load Bus/2 -> To Workspace I/1
  Single Phase Load Bus/3 -> To Workspace L/1
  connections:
  Phase/RConn1 -- Single Phase Load Bus/LConn1
  N/RConn1 -- Single Phase Load Bus/LConn2
  phase/RConn1 -- Single Phase Load Bus/RConn1
  n/RConn1 -- Single Phase Load Bus/RConn2

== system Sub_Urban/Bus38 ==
  Constant : Constant  Value=Ph
  Single Phase Load Bus : myLibrary/Single Phase Load Bus  SystemSampleTime=-1  Latency=0  AutoFrameSizeCalculation=off
  To Workspace I : ToWorkspace  VariableName=I38  SaveFormat=Structure With Time  SampleTime=-1
  To Workspace L : ToWorkspace  VariableName=Load25  SaveFormat=Structure With Time  SampleTime=-1
  To Workspace V : ToWorkspace  VariableName=Bus38  SaveFormat=Structure With Time  SampleTime=-1
  Phase : PMIOPort  Tag=PMCPort  Side=Left
  N : PMIOPort  Tag=PMCPort  Port=2  Side=Left
  phase : PMIOPort  Tag=PMCPort  Port=3  Side=Right
  n : PMIOPort  Tag=PMCPort  Port=4  Side=Right
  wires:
  Constant/1 -> Single Phase Load Bus/1
  Single Phase Load Bus/1 -> To Workspace V/1
  Single Phase Load Bus/2 -> To Workspace I/1
  Single Phase Load Bus/3 -> To Workspace L/1
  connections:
  Phase/RConn1 -- Single Phase Load Bus/LConn1
  N/RConn1 -- Single Phase Load Bus/LConn2
  phase/RConn1 -- Single Phase Load Bus/RConn1
  n/RConn1 -- Single Phase Load Bus/RConn2

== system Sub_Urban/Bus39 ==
  Three Phase Zero Bus : myLibrary/Three Phase Zero Bus  SystemSampleTime=-1  Latency=0  AutoFrameSizeCalculation=off
  To Workspace I : ToWorkspace  VariableName=I39  SaveFormat=Structure With Time  SampleTime=-1
  To Workspace V : ToWorkspace  VariableName=Bus39  SaveFormat=Structure With Time  SampleTime=-1
  A : PMIOPort  Tag=PMCPort  Side=Left
  B : PMIOPort  Tag=PMCPort  Port=2  Side=Left
  C : PMIOPort  Tag=PMCPort  Port=3  Side=Left
  N : PMIOPort  Tag=PMCPort  Port=4  Side=Left
  a : PMIOPort  Tag=PMCPort  Port=5  Side=Right
  b : PMIOPort  Tag=PMCPort  Port=6  Side=Right
  c : PMIOPort  Tag=PMCPort  Port=7  Side=Right
  n : PMIOPort  Tag=PMCPort  Port=8  Side=Right
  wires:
  Three Phase Zero Bus/1 -> To Workspace V/1
  Three Phase Zero Bus/2 -> To Workspace I/1
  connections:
  A/RConn1 -- Three Phase Zero Bus/LConn1
  B/RConn1 -- Three Phase Zero Bus/LConn2
  C/RConn1 -- Three Phase Zero Bus/LConn3
  N/RConn1 -- Three Phase Zero Bus/LConn4
  a/RConn1 -- Three Phase Zero Bus/RConn1
  b/RConn1 -- Three Phase Zero Bus/RConn2
  c/RConn1 -- Three Phase Zero Bus/RConn3
  n/RConn1 -- Three Phase Zero Bus/RConn4

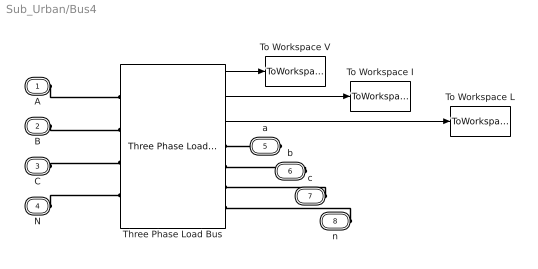
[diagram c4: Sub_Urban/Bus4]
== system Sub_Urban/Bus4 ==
  Three Phase Load Bus : myLibrary/Three Phase Load Bus  SystemSampleTime=-1  Latency=0  AutoFrameSizeCalculation=off
  To Workspace I : ToWorkspace  VariableName=I4  SaveFormat=Structure With Time  SampleTime=-1
  To Workspace L : ToWorkspace  VariableName=Load1  SaveFormat=Structure With Time  SampleTime=-1
  To Workspace V : ToWorkspace  VariableName=Bus4  SaveFormat=Structure With Time  SampleTime=-1
  A : PMIOPort  Tag=PMCPort  Side=Left
  B : PMIOPort  Tag=PMCPort  Port=2  Side=Left
  C : PMIOPort  Tag=PMCPort  Port=3  Side=Left
  N : PMIOPort  Tag=PMCPort  Port=4  Side=Left
  a : PMIOPort  Tag=PMCPort  Port=5  Side=Right
  b : PMIOPort  Tag=PMCPort  Port=6  Side=Right
  c : PMIOPort  Tag=PMCPort  Port=7  Side=Right
  n : PMIOPort  Tag=PMCPort  Port=8  Side=Right
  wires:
  Three Phase Load Bus/1 -> To Workspace V/1
  Three Phase Load Bus/2 -> To Workspace I/1
  Three Phase Load Bus/3 -> To Workspace L/1
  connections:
  N/RConn1 -- Three Phase Load Bus/LConn4
  C/RConn1 -- Three Phase Load Bus/LConn3
  n/RConn1 -- Three Phase Load Bus/RConn4
  B/RConn1 -- Three Phase Load Bus/LConn2
  A/RConn1 -- Three Phase Load Bus/LConn1
  b/RConn1 -- Three Phase Load Bus/RConn2
  c/RConn1 -- Three Phase Load Bus/RConn3
  a/RConn1 -- Three Phase Load Bus/RConn1

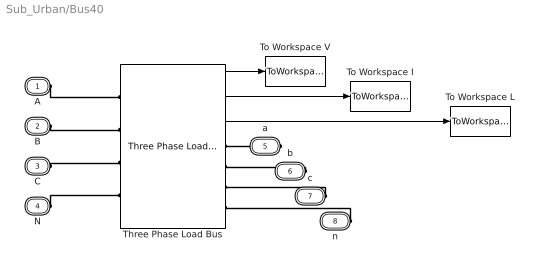
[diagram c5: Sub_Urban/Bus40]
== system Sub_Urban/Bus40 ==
  Three Phase Load Bus : myLibrary/Three Phase Load Bus  SystemSampleTime=-1  Latency=0  AutoFrameSizeCalculation=off
  To Workspace I : ToWorkspace  VariableName=I40  SaveFormat=Structure With Time  SampleTime=-1
  To Workspace L : ToWorkspace  VariableName=Load26  SaveFormat=Structure With Time  SampleTime=-1
  To Workspace V : ToWorkspace  VariableName=Bus40  SaveFormat=Structure With Time  SampleTime=-1
  A : PMIOPort  Tag=PMCPort  Side=Left
  B : PMIOPort  Tag=PMCPort  Port=2  Side=Left
  C : PMIOPort  Tag=PMCPort  Port=3  Side=Left
  N : PMIOPort  Tag=PMCPort  Port=4  Side=Left
  a : PMIOPort  Tag=PMCPort  Port=5  Side=Right
  b : PMIOPort  Tag=PMCPort  Port=6  Side=Right
  c : PMIOPort  Tag=PMCPort  Port=7  Side=Right
  n : PMIOPort  Tag=PMCPort  Port=8  Side=Right
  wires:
  Three Phase Load Bus/1 -> To Workspace V/1
  Three Phase Load Bus/2 -> To Workspace I/1
  Three Phase Load Bus/3 -> To Workspace L/1
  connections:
  N/RConn1 -- Three Phase Load Bus/LConn4
  C/RConn1 -- Three Phase Load Bus/LConn3
  n/RConn1 -- Three Phase Load Bus/RConn4
  B/RConn1 -- Three Phase Load Bus/LConn2
  A/RConn1 -- Three Phase Load Bus/LConn1
  b/RConn1 -- Three Phase Load Bus/RConn2
  c/RConn1 -- Three Phase Load Bus/RConn3
  a/RConn1 -- Three Phase Load Bus/RConn1

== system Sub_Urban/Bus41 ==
  Constant : Constant  Value=Ph
  Single Phase Load Bus : myLibrary/Single Phase Load Bus  SystemSampleTime=-1  Latency=0  AutoFrameSizeCalculation=off
  To Workspace I : ToWorkspace  VariableName=I41  SaveFormat=Structure With Time  SampleTime=-1
  To Workspace L : ToWorkspace  VariableName=Load27  SaveFormat=Structure With Time  SampleTime=-1
  To Workspace V : ToWorkspace  VariableName=Bus41  SaveFormat=Structure With Time  SampleTime=-1
  Phase : PMIOPort  Tag=PMCPort  Side=Left
  N : PMIOPort  Tag=PMCPort  Port=2  Side=Left
  phase : PMIOPort  Tag=PMCPort  Port=3  Side=Right
  n : PMIOPort  Tag=PMCPort  Port=4  Side=Right
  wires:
  Constant/1 -> Single Phase Load Bus/1
  Single Phase Load Bus/1 -> To Workspace V/1
  Single Phase Load Bus/2 -> To Workspace I/1
  Single Phase Load Bus/3 -> To Workspace L/1
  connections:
  Phase/RConn1 -- Single Phase Load Bus/LConn1
  N/RConn1 -- Single Phase Load Bus/LConn2
  phase/RConn1 -- Single Phase Load Bus/RConn1
  n/RConn1 -- Single Phase Load Bus/RConn2

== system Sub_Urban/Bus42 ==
  Constant : Constant  Value=Ph
  Single Phase Load Bus : myLibrary/Single Phase Load Bus  SystemSampleTime=-1  Latency=0  AutoFrameSizeCalculation=off
  To Workspace I : ToWorkspace  VariableName=I42  SaveFormat=Structure With Time  SampleTime=-1
  To Workspace L : ToWorkspace  VariableName=Load28  SaveFormat=Structure With Time  SampleTime=-1
  To Workspace V : ToWorkspace  VariableName=Bus42  SaveFormat=Structure With Time  SampleTime=-1
  Phase : PMIOPort  Tag=PMCPort  Side=Left
  N : PMIOPort  Tag=PMCPort  Port=2  Side=Left
  phase : PMIOPort  Tag=PMCPort  Port=3  Side=Right
  n : PMIOPort  Tag=PMCPort  Port=4  Side=Right
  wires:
  Constant/1 -> Single Phase Load Bus/1
  Single Phase Load Bus/1 -> To Workspace V/1
  Single Phase Load Bus/2 -> To Workspace I/1
  Single Phase Load Bus/3 -> To Workspace L/1
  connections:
  Phase/RConn1 -- Single Phase Load Bus/LConn1
  N/RConn1 -- Single Phase Load Bus/LConn2
  phase/RConn1 -- Single Phase Load Bus/RConn1
  n/RConn1 -- Single Phase Load Bus/RConn2

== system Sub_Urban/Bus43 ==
  Three Phase Zero Bus : myLibrary/Three Phase Zero Bus  SystemSampleTime=-1  Latency=0  AutoFrameSizeCalculation=off
  To Workspace I : ToWorkspace  VariableName=I43  SaveFormat=Structure With Time  SampleTime=-1
  To Workspace V : ToWorkspace  VariableName=Bus43  SaveFormat=Structure With Time  SampleTime=-1
  A : PMIOPort  Tag=PMCPort  Side=Left
  B : PMIOPort  Tag=PMCPort  Port=2  Side=Left
  C : PMIOPort  Tag=PMCPort  Port=3  Side=Left
  N : PMIOPort  Tag=PMCPort  Port=4  Side=Left
  a : PMIOPort  Tag=PMCPort  Port=5  Side=Right
  b : PMIOPort  Tag=PMCPort  Port=6  Side=Right
  c : PMIOPort  Tag=PMCPort  Port=7  Side=Right
  n : PMIOPort  Tag=PMCPort  Port=8  Side=Right
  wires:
  Three Phase Zero Bus/1 -> To Workspace V/1
  Three Phase Zero Bus/2 -> To Workspace I/1
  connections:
  A/RConn1 -- Three Phase Zero Bus/LConn1
  B/RConn1 -- Three Phase Zero Bus/LConn2
  C/RConn1 -- Three Phase Zero Bus/LConn3
  N/RConn1 -- Three Phase Zero Bus/LConn4
  a/RConn1 -- Three Phase Zero Bus/RConn1
  b/RConn1 -- Three Phase Zero Bus/RConn2
  c/RConn1 -- Three Phase Zero Bus/RConn3
  n/RConn1 -- Three Phase Zero Bus/RConn4

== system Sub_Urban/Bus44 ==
  Three Phase Zero Bus : myLibrary/Three Phase Zero Bus  SystemSampleTime=-1  Latency=0  AutoFrameSizeCalculation=off
  To Workspace I : ToWorkspace  VariableName=I44  SaveFormat=Structure With Time  SampleTime=-1
  To Workspace V : ToWorkspace  VariableName=Bus44  SaveFormat=Structure With Time  SampleTime=-1
  A : PMIOPort  Tag=PMCPort  Side=Left
  B : PMIOPort  Tag=PMCPort  Port=2  Side=Left
  C : PMIOPort  Tag=PMCPort  Port=3  Side=Left
  N : PMIOPort  Tag=PMCPort  Port=4  Side=Left
  a : PMIOPort  Tag=PMCPort  Port=5  Side=Right
  b : PMIOPort  Tag=PMCPort  Port=6  Side=Right
  c : PMIOPort  Tag=PMCPort  Port=7  Side=Right
  n : PMIOPort  Tag=PMCPort  Port=8  Side=Right
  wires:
  Three Phase Zero Bus/1 -> To Workspace V/1
  Three Phase Zero Bus/2 -> To Workspace I/1
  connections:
  A/RConn1 -- Three Phase Zero Bus/LConn1
  B/RConn1 -- Three Phase Zero Bus/LConn2
  C/RConn1 -- Three Phase Zero Bus/LConn3
  N/RConn1 -- Three Phase Zero Bus/LConn4
  a/RConn1 -- Three Phase Zero Bus/RConn1
  b/RConn1 -- Three Phase Zero Bus/RConn2
  c/RConn1 -- Three Phase Zero Bus/RConn3
  n/RConn1 -- Three Phase Zero Bus/RConn4

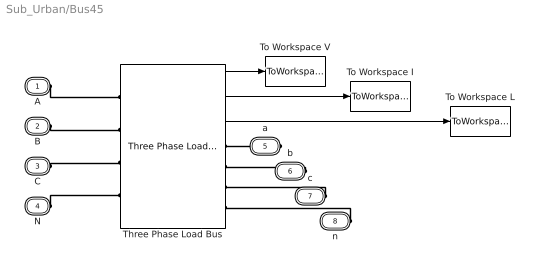
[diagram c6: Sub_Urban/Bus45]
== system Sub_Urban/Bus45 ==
  Three Phase Load Bus : myLibrary/Three Phase Load Bus  SystemSampleTime=-1  Latency=0  AutoFrameSizeCalculation=off
  To Workspace I : ToWorkspace  VariableName=I45  SaveFormat=Structure With Time  SampleTime=-1
  To Workspace L : ToWorkspace  VariableName=Load29  SaveFormat=Structure With Time  SampleTime=-1
  To Workspace V : ToWorkspace  VariableName=Bus45  SaveFormat=Structure With Time  SampleTime=-1
  A : PMIOPort  Tag=PMCPort  Side=Left
  B : PMIOPort  Tag=PMCPort  Port=2  Side=Left
  C : PMIOPort  Tag=PMCPort  Port=3  Side=Left
  N : PMIOPort  Tag=PMCPort  Port=4  Side=Left
  a : PMIOPort  Tag=PMCPort  Port=5  Side=Right
  b : PMIOPort  Tag=PMCPort  Port=6  Side=Right
  c : PMIOPort  Tag=PMCPort  Port=7  Side=Right
  n : PMIOPort  Tag=PMCPort  Port=8  Side=Right
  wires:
  Three Phase Load Bus/1 -> To Workspace V/1
  Three Phase Load Bus/2 -> To Workspace I/1
  Three Phase Load Bus/3 -> To Workspace L/1
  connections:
  N/RConn1 -- Three Phase Load Bus/LConn4
  C/RConn1 -- Three Phase Load Bus/LConn3
  n/RConn1 -- Three Phase Load Bus/RConn4
  B/RConn1 -- Three Phase Load Bus/LConn2
  A/RConn1 -- Three Phase Load Bus/LConn1
  b/RConn1 -- Three Phase Load Bus/RConn2
  c/RConn1 -- Three Phase Load Bus/RConn3
  a/RConn1 -- Three Phase Load Bus/RConn1

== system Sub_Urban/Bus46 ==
  Three Phase Zero Bus : myLibrary/Three Phase Zero Bus  SystemSampleTime=-1  Latency=0  AutoFrameSizeCalculation=off
  To Workspace I : ToWorkspace  VariableName=I46  SaveFormat=Structure With Time  SampleTime=-1
  To Workspace V : ToWorkspace  VariableName=Bus46  SaveFormat=Structure With Time  SampleTime=-1
  A : PMIOPort  Tag=PMCPort  Side=Left
  B : PMIOPort  Tag=PMCPort  Port=2  Side=Left
  C : PMIOPort  Tag=PMCPort  Port=3  Side=Left
  N : PMIOPort  Tag=PMCPort  Port=4  Side=Left
  a : PMIOPort  Tag=PMCPort  Port=5  Side=Right
  b : PMIOPort  Tag=PMCPort  Port=6  Side=Right
  c : PMIOPort  Tag=PMCPort  Port=7  Side=Right
  n : PMIOPort  Tag=PMCPort  Port=8  Side=Right
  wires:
  Three Phase Zero Bus/1 -> To Workspace V/1
  Three Phase Zero Bus/2 -> To Workspace I/1
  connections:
  A/RConn1 -- Three Phase Zero Bus/LConn1
  B/RConn1 -- Three Phase Zero Bus/LConn2
  C/RConn1 -- Three Phase Zero Bus/LConn3
  N/RConn1 -- Three Phase Zero Bus/LConn4
  a/RConn1 -- Three Phase Zero Bus/RConn1
  b/RConn1 -- Three Phase Zero Bus/RConn2
  c/RConn1 -- Three Phase Zero Bus/RConn3
  n/RConn1 -- Three Phase Zero Bus/RConn4

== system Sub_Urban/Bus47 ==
  Constant : Constant  Value=Ph
  Single Phase Load Bus : myLibrary/Single Phase Load Bus  SystemSampleTime=-1  Latency=0  AutoFrameSizeCalculation=off
  To Workspace I : ToWorkspace  VariableName=I47  SaveFormat=Structure With Time  SampleTime=-1
  To Workspace L : ToWorkspace  VariableName=Load30  SaveFormat=Structure With Time  SampleTime=-1
  To Workspace V : ToWorkspace  VariableName=Bus47  SaveFormat=Structure With Time  SampleTime=-1
  Phase : PMIOPort  Tag=PMCPort  Side=Left
  N : PMIOPort  Tag=PMCPort  Port=2  Side=Left
  phase : PMIOPort  Tag=PMCPort  Port=3  Side=Right
  n : PMIOPort  Tag=PMCPort  Port=4  Side=Right
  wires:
  Constant/1 -> Single Phase Load Bus/1
  Single Phase Load Bus/1 -> To Workspace V/1
  Single Phase Load Bus/2 -> To Workspace I/1
  Single Phase Load Bus/3 -> To Workspace L/1
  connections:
  Phase/RConn1 -- Single Phase Load Bus/LConn1
  N/RConn1 -- Single Phase Load Bus/LConn2
  phase/RConn1 -- Single Phase Load Bus/RConn1
  n/RConn1 -- Single Phase Load Bus/RConn2

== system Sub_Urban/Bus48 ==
  Constant : Constant  Value=Ph
  Single Phase Load Bus : myLibrary/Single Phase Load Bus  SystemSampleTime=-1  Latency=0  AutoFrameSizeCalculation=off
  To Workspace I : ToWorkspace  VariableName=I48  SaveFormat=Structure With Time  SampleTime=-1
  To Workspace L : ToWorkspace  VariableName=Load31  SaveFormat=Structure With Time  SampleTime=-1
  To Workspace V : ToWorkspace  VariableName=Bus48  SaveFormat=Structure With Time  SampleTime=-1
  Phase : PMIOPort  Tag=PMCPort  Side=Left
  N : PMIOPort  Tag=PMCPort  Port=2  Side=Left
  phase : PMIOPort  Tag=PMCPort  Port=3  Side=Right
  n : PMIOPort  Tag=PMCPort  Port=4  Side=Right
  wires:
  Constant/1 -> Single Phase Load Bus/1
  Single Phase Load Bus/1 -> To Workspace V/1
  Single Phase Load Bus/2 -> To Workspace I/1
  Single Phase Load Bus/3 -> To Workspace L/1
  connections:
  Phase/RConn1 -- Single Phase Load Bus/LConn1
  N/RConn1 -- Single Phase Load Bus/LConn2
  phase/RConn1 -- Single Phase Load Bus/RConn1
  n/RConn1 -- Single Phase Load Bus/RConn2
